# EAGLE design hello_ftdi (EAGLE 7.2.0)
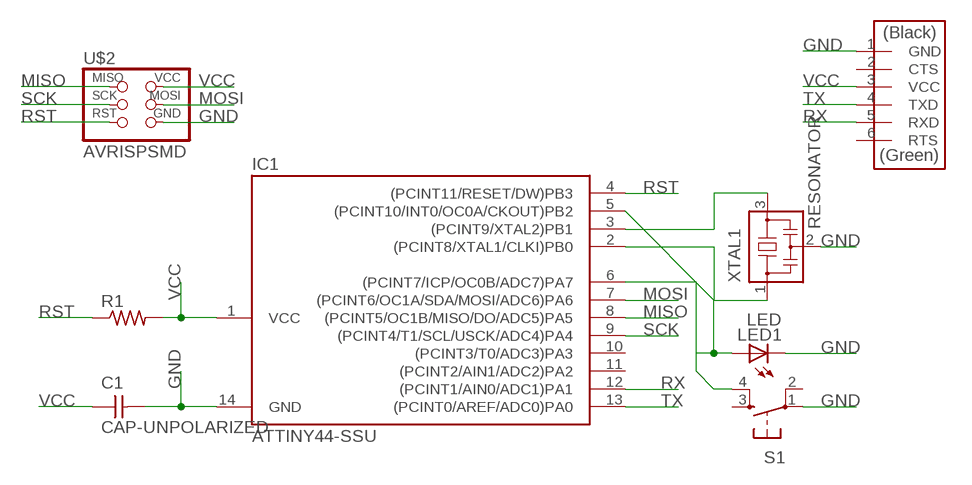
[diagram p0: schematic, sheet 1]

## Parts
C1  CAP-UNPOLARIZED  [C1206]
IC1  ATTINY44-SSU  [SOIC14]
LED1  LED  [LED1206]
R1  RES-US1206  [R1206]
S1  6MM_SWITCH6MM_SWITCH  [6MM_SWITCH]
U$2  AVRISPSMD  [2X03SMD]
U$3  FTDI-SMD-HEADER  [1X06SMD]
XTAL1  RESONATOR  [EFOBM]

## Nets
GND: C1.2 IC1.14(GND) LED1.2(C) S1.1(P) U$2.6(GND) U$3.1(GND) XTAL1.2
MISO: IC1.8((PCINT5/OC1B/MISO/DO/ADC5)PA5) U$2.1(MISO)
MOSI: IC1.7((PCINT6/OC1A/SDA/MOSI/ADC6)PA6) U$2.4(MOSI)
N$1: IC1.5((PCINT10/INT0/OC0A/CKOUT)PB2) LED1.1(A)
N$3: IC1.6((PCINT7/ICP/OC0B/ADC7)PA7) S1.4(S1)
N$4: IC1.3((PCINT9/XTAL2)PB1) XTAL1.3
N$5: IC1.2((PCINT8/XTAL1/CLKI)PB0) XTAL1.1
RST: IC1.4((PCINT11/RESET/DW)PB3) R1.1 U$2.5(RST)
RX: IC1.12((PCINT1/AIN0/ADC1)PA1) U$3.5(RXD)
SCK: IC1.9((PCINT4/T1/SCL/USCK/ADC4)PA4) U$2.3(SCK)
TX: IC1.13((PCINT0/AREF/ADC0)PA0) U$3.4(TXD)
VCC: C1.1 IC1.1(VCC) R1.2 U$2.2(VCC) U$3.3(VCC)
Unconnected: IC1.10((PCINT3/T0/ADC3)PA3) IC1.11((PCINT2/AIN1/ADC2)PA2) S1.2(P1) S1.3(S) U$3.2(CTS) U$3.6(RTS)

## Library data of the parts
C1 = fab:CAP-UNPOLARIZED
IC1 = fab:ATTINY44
LED1 = fab:LED: LED
R1 = fab:RES-US: Resistor (US Symbol)
S1 = fab:6MM_SWITCH: OMRON SWITCH
U$2 = fab:AVRISP
U$3 = fab:FTDI-SMD-HEADER
XTAL1 = fab:RESONATOR

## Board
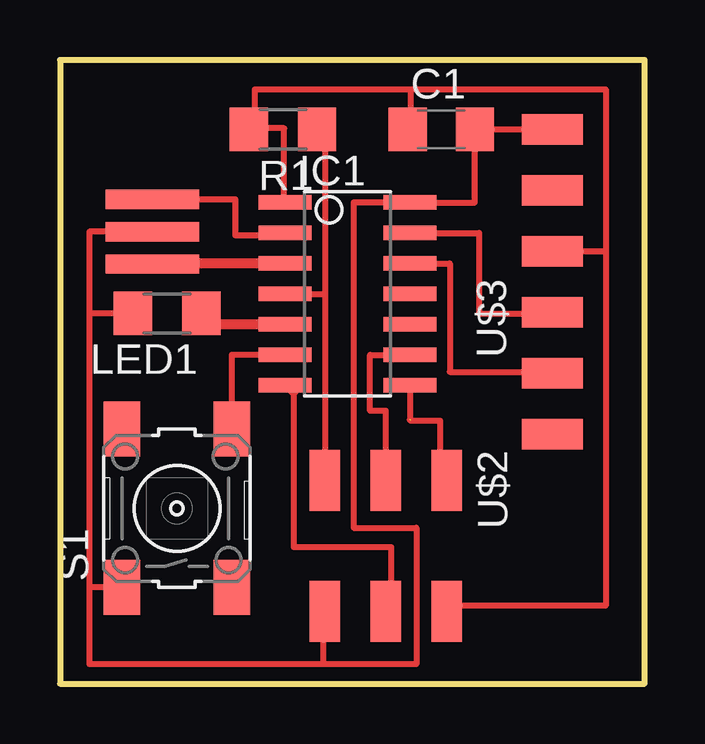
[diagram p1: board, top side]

Size 24.38 x 26.01 mm. Coordinates in mm from the lower left corner, seen from the top.
Outline: 0,0 24.38,0 24.38,26.01 0,26.01 0,0
Copper layers 1+16: Top 0.035mm / dielectric 1.5mm / Bottom 0.035mm
Design rules "fablab_17mils": minimum track width 10mil, minimum drill 0.8mm, track to track 17mil, track to pad 17mil, pad to pad 17mil, via to via 17mil, smd to smd 17mil, copper to edge 16mil, drill to drill 16mil, minimum pad ring 0.8mm, minimum via ring 0.8mm, stop-mask expansion 4mil, vias tented up to drill 0mil, thermal gap 1mm

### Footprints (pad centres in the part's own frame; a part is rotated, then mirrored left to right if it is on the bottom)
C1206 = smd 1.6 x 1.8: 1 -1.4,0; 2 1.4,0
SOIC14 = smd 0.61 x 2.21: 1 -3.81,-2.603; 2 -2.54,-2.603; 3 -1.27,-2.603; 4 0,-2.603; 5 1.27,-2.603; 6 2.54,-2.603; 7 3.81,-2.603; 8 3.81,2.603; 9 2.54,2.603; 10 1.27,2.603; 11 0,2.603; 12 -1.27,2.603; 13 -2.54,2.603; 14 -3.81,2.603
LED1206 = smd 1.6 x 1.803: 1 -1.422,0; 2 1.422,0
R1206 = smd 1.6 x 1.803: 1 -1.422,0; 2 1.422,0
6MM_SWITCH = smd 2.286 x 1.524: 1 -3.302,2.286; 2 3.302,2.286; 3 -3.302,-2.286; 4 3.302,-2.286
2X03SMD = smd 2.54 x 1.27: 1 -2.54,2.54; 2 2.92,2.54; 3 -2.54,0; 4 2.92,0; 5 -2.54,-2.54; 6 2.92,-2.54
1X06SMD = smd 2.54 x 1.27: 1 0,6.35; 2 0,3.81; 3 0,1.27; 4 0,-1.27; 5 0,-3.81; 6 0,-6.35
EFOBM = smd 0.8 x 3.9: 1 -1.35,0; 2 0,0; 3 1.35,0

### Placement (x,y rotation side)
C1  1uF  [C1206]  15.9,23.11 0 top
IC1  11.99,16.26 270 top
LED1  4.47,15.44 180 top
R1  10k  [R1206]  9.3,23.11 180 top
S1  4.88,7.32 90 top
U$2  13.59,5.94 270 top
U$3  20.52,16.76 0 top
XTAL1  3.86,18.85 270 top

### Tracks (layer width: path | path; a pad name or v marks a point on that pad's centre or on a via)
GND
  Top 0.254: U$3.1 C1.2 17.3,20.07 IC1.14 12.24,20.07 12.24,6.5 14.86,6.5 14.86,0.81 10.97,0.81 | XTAL1.2 1.22,18.85 1.22,15.44 | 1.22,15.44 1.22,4.01 | 1.22,4.01 1.22,0.81 10.97,0.81 | U$2.6 11.05,3.25 10.97,3.25 10.97,0.81 | LED1.2 1.22,15.44 | S1.1 1.22,4.01
MISO  (1 unrouted)
  Top 0.254: IC1.8 14.59,11.01 | 14.63,10.97 15.85,10.97 15.85,9.09
  Top 0.406: 15.85,9.09 arc90 U$2.1
MOSI
  Top 0.254: 13.82,3.58 13.82,5.69 9.75,5.69 9.75,12.19
  Top 0.406: U$2.4 13.82,3.58 | 9.75,12.19 9.5,12.45 IC1.7
N$1
  Top 0.406: IC1.5 5.89,14.99 LED1.1
N$3
  Top 0.254: IC1.6 7.16,13.72 S1.4
N$4
  Top 0.406: IC1.3 3.86,17.53 XTAL1.3
N$5
  Top 0.254: 9.13,18.69 7.32,18.69 7.32,20.2 XTAL1.1
  Top 0.406: IC1.2 9.13,18.69
RST
  Top 0.254: 10.97,8.23 U$2.5 11.05,16.26 | R1.1 11.05,22.78 11.05,16.26 | IC1.4 11.05,16.26
  Top 0.406: R1.1 10.97,23.11 | U$2.5 arc-90 10.97,8.23
RX
  Top 0.254: IC1.12 16.26,17.53 16.26,13.01 21.34,13.01
  Top 0.406: 21.34,13.01 U$3.5
SCK
  Top 0.254: U$2.3 13.59,11.38 12.93,11.38 12.93,13.72 IC1.9
TX
  Top 0.254: IC1.13 17.48,18.8 17.48,15.44 21.34,15.44
  Top 0.406: 21.34,15.44 U$3.4
VCC
  Top 0.254: 9.35,20.07 9.35,23.16 8.13,23.16 8.13,24.79 14.63,24.79 | 14.63,24.79 22.76,24.79 22.76,18.03 | 14.63,23.11 14.63,24.79 | 22.76,18.03 22.76,3.25 16.31,3.25 | U$3.3 22.76,18.03
  Top 0.406: IC1.1 9.35,20.07 | 8.13,23.16 7.82,23.16 R1.2 | C1.1 14.63,23.11 | 16.31,3.25 U$2.2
